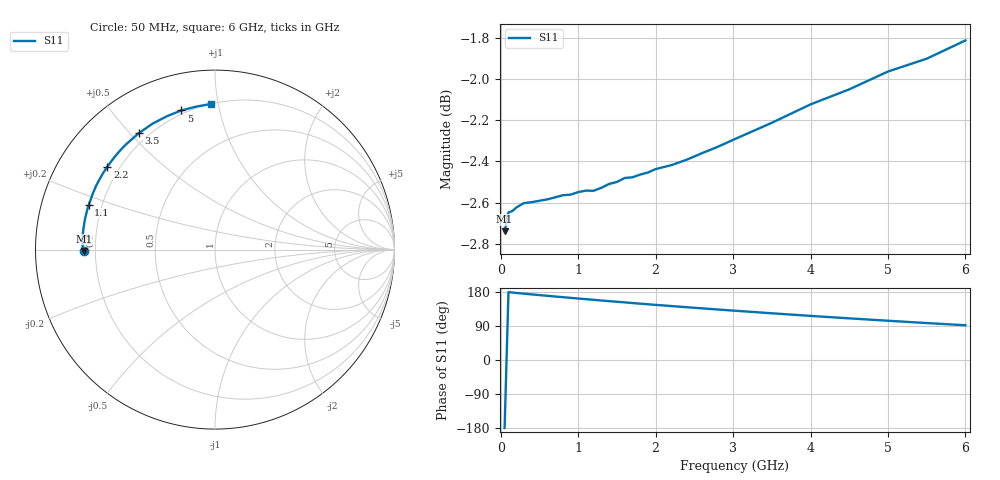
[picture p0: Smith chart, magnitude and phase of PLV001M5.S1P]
! Infineon Technologies  Discrete & RF Semiconductors
! BAR 64-04W /-05W /-06W
! Si PIN Diode in SOT323
! IF = 1.5 mA
! S-Parameters:  October  2008
# GHz  S  MA  R  50
!  f  S11
! GHz  MAG  ANG
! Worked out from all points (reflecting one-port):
!   34 points, 50 MHz to 6 GHz, reference 50 ohm
!   lowest |S11| = -2.7 dB at 50 MHz (marker M1), VSWR 6.39, Z = 7.82 - j0.255 ohm
!   phase of S11 starts at -179 deg and turns -89 deg over the sweep
!   S11 on the Smith chart (normalised r, x): 50 MHz: 0.16, -0.01; 1.1 GHz: 0.15, +0.17; 2.2 GHz: 0.15, +0.33; 3.5 GHz: 0.16, +0.53; 5 GHz: 0.18, +0.77; 6 GHz: 0.20, +0.95
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0.05  0.7295 -179.4
0.1  0.7372 179.2
0.2  0.7392 177.0
0.25  0.7402 176.1
0.3  0.7411 175.1
0.4  0.7415 173.1
0.5  0.7421 171.3
0.6  0.7427 169.4
0.8  0.7444 165.8
0.9  0.7446 164.0
1  0.7457 162.3
1.1  0.7463 160.5
1.4  0.7491 155.3
1.6  0.7516 152.1
1.7  0.7519 150.3
1.8  0.753 148.7
2  0.7554 145.5
2.2  0.757 142.4
2.4  0.7593 139.3
2.6  0.7621 136.3
2.8  0.7648 133.3
3  0.7678 130.4
3.5  0.7752 123.3
4  0.7832 116.4
4.5  0.7898 109.9
5  0.7977 103.6
5.5  0.8035 97.5
6  0.8117 91.7
